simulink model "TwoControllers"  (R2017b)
settings: Solver=ode15s  StartTime=0.0  StopTime=6000  MaxStep=0.1  RelTol=1e-5
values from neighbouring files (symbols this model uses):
  d = Tin_c(i)    [ActiveConstraints.m]    (also in Main.m = 293.15)
  Kc_c = 0    [ActiveConstraints.m]    (also in Main.m = -0.055)
  Kc_h = 0.0803    [ActiveConstraints.m]    (also in Main.m)
  N = 10    [ActiveConstraints.m]    (also in Main.m; SRC_ODE.m = p(8))
  p = [rho_c; rho_h; Tin_h; U; A; cp_c; cp_h;N;F_c_max;F_h_max]    [ActiveConstraints.m]    (also in Main.m)
  tauI_c = 1    [ActiveConstraints.m]    (also in Main.m = 74)
  tauI_h = 86    [ActiveConstraints.m]    (also in Main.m)
  ThSP = x0(end)    [ActiveConstraints.m]    (also in Main.m)
  ThSP2 = ThSP+1    [Main.m]
  x0 = [Tc0; Th0]    [ActiveConstraints.m]    (also in Main.m; col_obj.m = 0.5*ones(1,82)'; Simulate1Col.m = x; Simulate1Col_OL.m = x)
  z_c = F_c/F_c_max    (= 1)    [ActiveConstraints.m]    (also in Main.m = 0.5; SRC_ODE.m = u(1))
  z_h = F_h./F_h_max    [ActiveConstraints.m]    (also in Main.m = 1; SRC_ODE.m = u(2))
undefined symbols (not defined in the file or in its folder): SRC_ODE
libraries: simulink x2

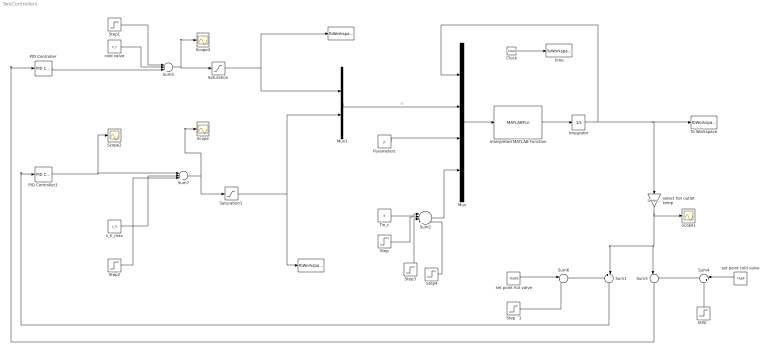
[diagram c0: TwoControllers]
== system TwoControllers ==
  " " : ToWorkspace  VariableName=u1  SampleTime=-1
  "  " : ToWorkspace  VariableName=u2  SampleTime=-1
  Clock : Clock
  Integrator : Integrator  InitialCondition=x0'
  Interpreted MATLAB Function : MATLABFcn  MATLABFcn=SRC_ODE(u(1:20),u(21:22),u(23:32),u(33))  OutputDimensions=20  Output1D=off
  Mux : Mux
  Mux1 : Mux  Inputs=2
  PID Controller : simulink/Continuous/PID Controller  Controller=PI  TimeDomain=Continuous-time  SampleTime=-1  IntegratorMethod=Forward Euler  FilterMethod=Forward Euler  Form=Parallel  UseFilter=on  ControllerParametersSource=internal  P=Kc_c  I=Kc_c/tauI_c  D=0  N=100  InitialConditionSource=internal  InitialConditionForIntegrator=0  InitialConditionForFilter=0  ExternalReset=none  IgnoreLimit=on  ZeroCross=off  LimitOutput=off  UpperSaturationLimit=1  LowerSaturationLimit=0  LinearizeAsGain=on  AntiWindupMode=back-calculation  Kb=1  TrackingMode=off  Kt=1  PParamMin=[]  PParamMax=[]  IParamMin=[]  IParamMax=[]  DParamMin=[]  DParamMax=[]  NParamMin=[]  NParamMax=[]  KbParamMin=[]  KbParamMax=[]  KtParamMin=[]  KtParamMax=[]  POutMin=[]  POutMax=[]  IOutMin=[]  IOutMax=[]  DOutMin=[]  DOutMax=[]  NOutMin=[]  NOutMax=[]  KbOutMin=[]  KbOutMax=[]  KtOutMin=[]  KtOutMax=[]  IntegratorOutMin=[]  IntegratorOutMax=[]  FilterOutMin=[]  FilterOutMax=[]  SumOutMin=[]  SumOutMax=[]  SumI1OutMin=[]  SumI1OutMax=[]  SumI2OutMin=[]  SumI2OutMax=[]  SumI3OutMin=[]  SumI3OutMax=[]  SumDOutMin=[]  SumDOutMax=[]  SaturationOutMin=[]  SaturationOutMax=[]  IntegratorContinuousStateAttributes=''  IntegratorStateMustResolveToSignalObject=off  IntegratorRTWStateStorageClass=Auto  FilterContinuousStateAttributes=''  FilterStateMustResolveToSignalObject=off  FilterRTWStateStorageClass=Auto  DifferentiatorICPrevScaledInput=0  DifferentiatorOutMin=[]  DifferentiatorOutMax=[]  InitialConditionSetting=State (most efficient)  FilterDiffOutCoefMin=[]  FilterDiffOutCoefMax=[]  SumDenOutMin=[]  SumDenOutMax=[]  SumNumOutMin=[]  SumNumOutMax=[]  ReciprocalOutMin=[]  ReciprocalOutMax=[]  DivideOutMin=[]  DivideOutMax=[]  TunerSelectOption=Transfer Function Based (PID Tuner App)
  PID Controller1 : simulink/Continuous/PID Controller  Controller=PI  TimeDomain=Continuous-time  SampleTime=-1  IntegratorMethod=Forward Euler  FilterMethod=Forward Euler  Form=Parallel  UseFilter=on  ControllerParametersSource=internal  P=Kc_h  I=Kc_h/tauI_h  D=0  N=100  InitialConditionSource=internal  InitialConditionForIntegrator=0  InitialConditionForFilter=0  ExternalReset=none  LimitOutput=off  UpperSaturationLimit=0  LowerSaturationLimit=-1  LinearizeAsGain=on  AntiWindupMode=back-calculation  Kb=1  TrackingMode=off  Kt=1  PParamMin=[]  PParamMax=[]  IParamMin=[]  IParamMax=[]  DParamMin=[]  DParamMax=[]  NParamMin=[]  NParamMax=[]  KbParamMin=[]  KbParamMax=[]  KtParamMin=[]  KtParamMax=[]  POutMin=[]  POutMax=[]  IOutMin=[]  IOutMax=[]  DOutMin=[]  DOutMax=[]  NOutMin=[]  NOutMax=[]  KbOutMin=[]  KbOutMax=[]  KtOutMin=[]  KtOutMax=[]  IntegratorOutMin=[]  IntegratorOutMax=[]  FilterOutMin=[]  FilterOutMax=[]  SumOutMin=[]  SumOutMax=[]  SumI1OutMin=[]  SumI1OutMax=[]  SumI2OutMin=[]  SumI2OutMax=[]  SumI3OutMin=[]  SumI3OutMax=[]  SumDOutMin=[]  SumDOutMax=[]  SaturationOutMin=[]  SaturationOutMax=[]  IntegratorContinuousStateAttributes=''  IntegratorStateMustResolveToSignalObject=off  IntegratorRTWStateStorageClass=Auto  FilterContinuousStateAttributes=''  FilterStateMustResolveToSignalObject=off  FilterRTWStateStorageClass=Auto  DifferentiatorICPrevScaledInput=0  DifferentiatorOutMin=[]  DifferentiatorOutMax=[]  InitialConditionSetting=State (most efficient)  FilterDiffOutCoefMin=[]  FilterDiffOutCoefMax=[]  SumDenOutMin=[]  SumDenOutMax=[]  SumNumOutMin=[]  SumNumOutMax=[]  ReciprocalOutMin=[]  ReciprocalOutMax=[]  DivideOutMin=[]  DivideOutMax=[]  TunerSelectOption=Transfer Function Based (PID Tuner App)
  Parameters : Constant  Value=p
  Saturation : Saturate  UpperLimit=1  LowerLimit=0
  Saturation1 : Saturate  UpperLimit=1  LowerLimit=0
  Scope{,1..2,4} (4 alike) : Scope
  Step : Step  Time=200  After=2  SampleTime=0
  "Step   " : Step  Time=50  After=0  SampleTime=0
  Step   1 : Step  Time=50  After=0  SampleTime=0
  Step1 : Step  Time=0  After=0  SampleTime=0
  Step2 : Step  Time=100  After=-0.1  SampleTime=0
  Step3 : Step  Time=2000  After=4  SampleTime=0
  Step4 : Step  Time=4000  After=0  SampleTime=0
  Sum1 : Sum  Inputs=+-|
  Sum2 : Sum  Inputs=|++++
  Sum3 : Sum  Inputs=|-+
  Sum4 : Sum  Inputs=|++
  Sum5 : Sum  Inputs=+++|
  Sum6 : Sum  Inputs=|++
  Sum7 : Sum  Inputs=|+++
  Tin_c : Constant  Value=d
  To Workspace : ToWorkspace  VariableName=y  SampleTime=-1
  cold valve : Constant  Value=z_c
  select hot outlet temp : Gain  Gain=[zeros(1,2*N-1),1]  Multiplication=Matrix(K*u)
  set point cold valve : Constant  Value=ThSP
  set point hot valve : Constant  Value=ThSP2
  time : ToWorkspace  VariableName=t  SampleTime=-1
  z_h_max : Constant  Value=z_h
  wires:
  Interpreted MATLAB Function/1 -> Integrator/1
  Integrator/1 -> Mux/1, select hot outlet temp/1, To Workspace/1
  Mux/1 -> Interpreted MATLAB Function/1
  Clock/1 -> time/1
  Mux1/1 -> Mux/2  "u"
  Parameters/1 -> Mux/3
  Tin_c/1 -> Sum2/1
  Step/1 -> Sum2/2
  Sum2/1 -> Mux/4
  Sum4/1 -> Sum3/2
  "Step   "/1 -> Sum4/2
  set point cold valve/1 -> Sum4/1
  Sum3/1 -> PID Controller/1
  z_h_max/1 -> Sum7/2
  Saturation/1 -> Mux1/1, " "/1
  Sum5/1 -> Scope4/1, Saturation/1
  Sum7/1 -> Saturation1/1, Scope/1
  Saturation1/1 -> Mux1/2, "  "/1
  PID Controller/1 -> Sum5/3
  cold valve/1 -> Sum5/2
  Step1/1 -> Sum5/1
  Step2/1 -> Sum7/3
  Step3/1 -> Sum2/3
  Step4/1 -> Sum2/4
  select hot outlet temp/1 -> Sum1/2, Sum3/1, Scope1/1
  Sum6/1 -> Sum1/1
  set point hot valve/1 -> Sum6/1
  Step   1/1 -> Sum6/2
  PID Controller1/1 -> Sum7/1, Scope2/1
  Sum1/1 -> PID Controller1/1
